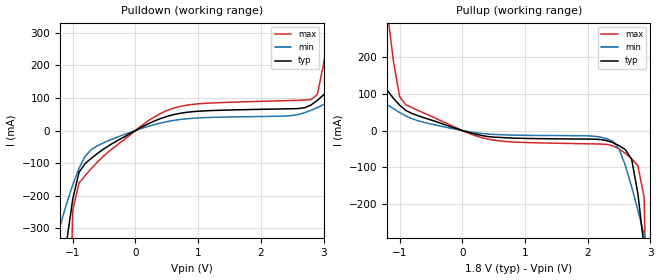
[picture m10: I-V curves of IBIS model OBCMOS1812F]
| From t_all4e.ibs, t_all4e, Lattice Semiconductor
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|   OBCMOS1812F
[Model]   OBCMOS1812F
Model_type   Output
Polarity   Non-Inverting
C_comp   2pF   2pF   2pF
[Temperature Range]   25.0000   125.0000   -40.0000
[Voltage Range]   1.8000V   1.7000V   1.9000V
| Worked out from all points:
|   slope of the pulldown table from 0 to 0.27 V, typ, clamps not added: 10.3 ohm
|   slope of the pullup table from 0 to 0.27 V, typ, clamps not added: 22.3 ohm
[Pulldown]
|voltage   I(typ)   I(min)   I(max)
-1.8V     -1.596A    -714.9mA   -13.05A
-1.3V     -679.3mA   -358.9mA   -4.192A
-1.2V     -506.1mA   -291.1mA   -2.535A
-1.1V     -345.4mA   -226mA     -1.059A
-900mV    -127.9mA   -116.1mA   -161mA
-700mV    -84.45mA   -57.73mA   -115.9mA
-500mV    -55.75mA   -36.94mA   -76.76mA
700mV     52.35mA    33.46mA    73.29mA
2.8V      78.24mA    61.92mA    94.92mA
2.9V      91.99mA    70.26mA    110.1mA
3.1V      129.9mA    89.53mA    339.1mA
3.6V      248.9mA    151.8mA    1.143A
[Pullup]
|voltage   I(typ)   I(min)   I(max)
-1.8V     259.9mA    149.3mA    1.315A
-1.2V     110.2mA    71.04mA    332.9mA
-1V       69.11mA    49.05mA    92.12mA
-800mV    46.28mA    32.02mA    62.08mA
400mV     -16.33mA   -9.277mA   -22.98mA
2.4V      -32.79mA   -29.21mA   -41.58mA
2.5V      -41.01mA   -50.46mA   -49.85mA
2.7V      -77.99mA   -153.2mA   -77.44mA
2.8V      -172mA     -217.5mA   -95.93mA
2.9V      -320.9mA   -284.8mA   -182.4mA
3V        -488.7mA   -353.9mA   -1.018A
3.6V      -1.584A    -784.5mA   -11.23A
[Ramp]
| variable   typ   min   max
dV/dt_r   0.5814/0.2955ns   0.3828/0.4907ns   0.8196/0.1700ns
dV/dt_f   0.8966/0.7099ns   0.7619/1.5741ns   0.9962/0.3022ns
